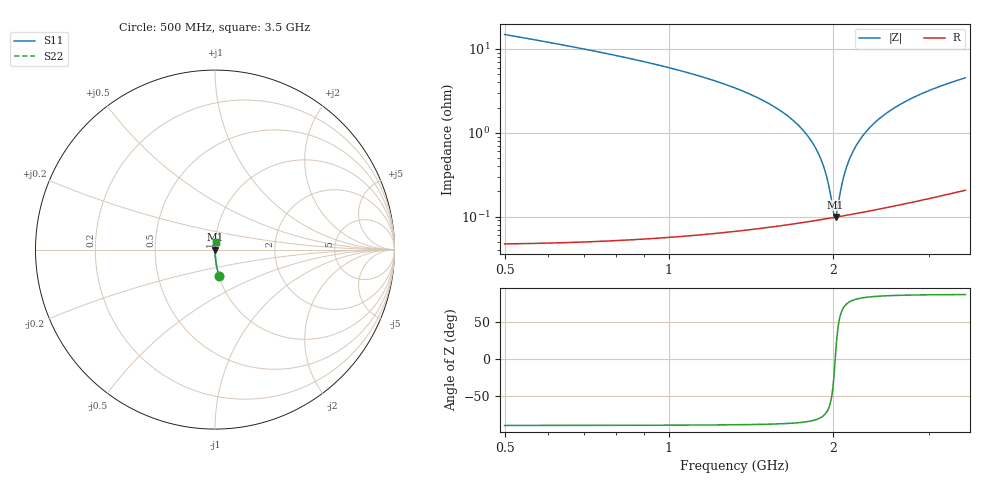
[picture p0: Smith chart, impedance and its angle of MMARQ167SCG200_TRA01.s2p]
! MMARQ167SCG200_TRA01  S-PARAMETER MODEL  ( General Type )
! Model Generated by TAIYO YUDEN Corporation (http://www.ty-top.com)
! Version 1.0
! TAIYO YUDEN Control No. 160201
! Copyright(c) 2016 TAIYO YUDEN CO.,LTD. All Rights Reserved.
! Product Description (link to TY-COMPAS)
! https://ds.yuden.co.jp/TYCOMPAS/or/detail?pn=MMARQ167SCG200JTRA01&u=M
! Products Name : Multilayer Ceramic Capacitors
! Characteristics :
!  Capacitance : 20 pF , Rated Voltage : 250V , TCC : CG / C0G
!  Case Size : 1.6 x 0.8 / 0.063 x 0.031 [mm/inch] , Thickness : 0.7 / 0.028 [mm/inch]
!  (Conditions: Temperature = 25 degC , DC Bias Current/Voltage = 0A / 0V)
! External Node Assignments :
!  1  o---| |---o  2
! GND o---------o GND
! Frequency Range : 500MHz  -  3500MHz  [ 401 STEP ]
# MHz S RI R 50
! Freq[MHz].  S11 Real  S11 Imag  S21 Real  S21 Imag  S12 Real  S12 Imag  S22 Real  S22 Imag
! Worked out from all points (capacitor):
!   401 points, 500 MHz to 3.5 GHz, reference 50 ohm
!   read as one part in series: C = 20 pF near 515 MHz
!   lowest |Z| = 98.9 mohm at 2.022 GHz (marker M1)
!   series resonance near 2.02 GHz, so ESL is about 310 pH
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500  0.0222 -0.1459  0.9778 0.1459  0.9778 0.1459  0.0222 -0.1459
1002.5  0.00412 -0.0595  0.9959 0.0595  0.9959 0.0595  0.00412 -0.0595
1505  0.00129 -0.0234  0.9987 0.0234  0.9987 0.0234  0.00129 -0.0234
1700  0.00101 -0.0136  0.999 0.0136  0.999 0.0136  0.00101 -0.0136
1842.5  0.000941 -0.00723  0.9991 0.00723  0.9991 0.00723  0.000941 -0.00723
1895  0.000941 -0.00501  0.9991 0.00501  0.9991 0.00501  0.000941 -0.00501
1932.5  0.000947 -0.00347  0.9991 0.00347  0.9991 0.00347  0.000947 -0.00347
1962.5  0.000956 -0.00226  0.999 0.00226  0.999 0.00226  0.000956 -0.00226
2000  0.000971 -0.000778  0.999 0.000778  0.999 0.000778  0.000971 -0.000778
2015  0.000979 -0.000192  0.999 0.000192  0.999 0.000192  0.000979 -0.000192
2022.5  0.000983 9.93e-05  0.999 -9.93e-05  0.999 -9.93e-05  0.000983 9.93e-05
2037.5  0.000992 0.000679  0.999 -0.000679  0.999 -0.000679  0.000992 0.000679
2067.5  0.00101 0.00183  0.999 -0.00183  0.999 -0.00183  0.00101 0.00183
2097.5  0.00103 0.00296  0.999 -0.00296  0.999 -0.00296  0.00103 0.00296
2135  0.00106 0.00435  0.9989 -0.00435  0.9989 -0.00435  0.00106 0.00435
2180  0.00111 0.00599  0.9989 -0.00599  0.9989 -0.00599  0.00111 0.00599
2240  0.00117 0.00812  0.9988 -0.00812  0.9988 -0.00812  0.00117 0.00812
2315  0.00127 0.0107  0.9987 -0.0107  0.9987 -0.0107  0.00127 0.0107
2502.5  0.00156 0.0169  0.9984 -0.0169  0.9984 -0.0169  0.00156 0.0169
2720  0.00198 0.0236  0.998 -0.0236  0.998 -0.0236  0.00198 0.0236
3005  0.00266 0.0319  0.9973 -0.0319  0.9973 -0.0319  0.00266 0.0319
3500  0.00409 0.045  0.9959 -0.045  0.9959 -0.045  0.00409 0.045
